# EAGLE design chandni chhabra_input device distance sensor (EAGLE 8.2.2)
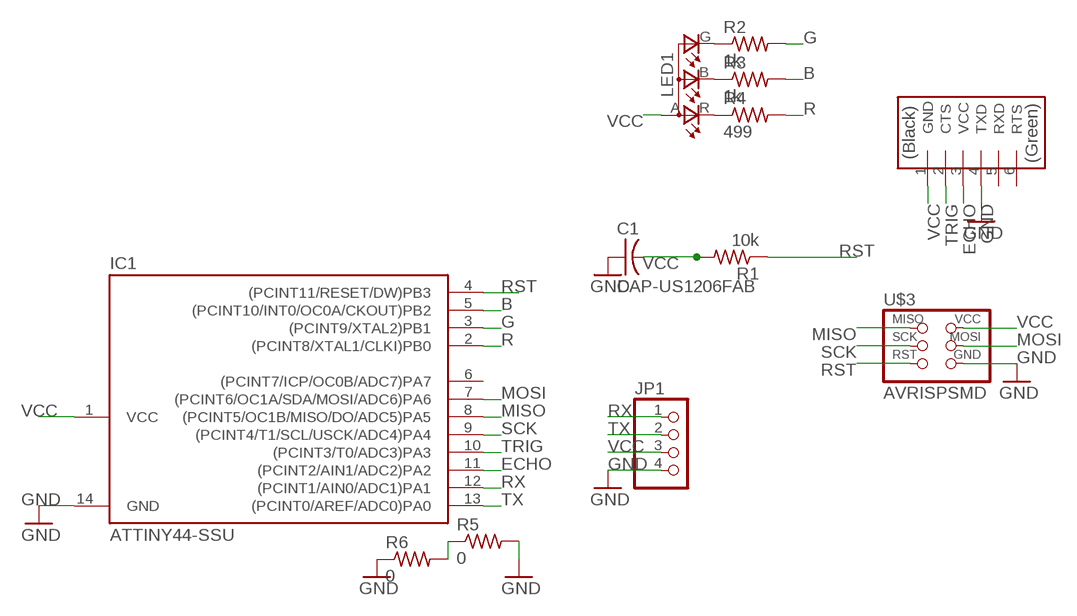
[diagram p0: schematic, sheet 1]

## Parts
C1  CAP-US1206FAB  [C1206FAB]
IC1  ATTINY44-SSU  [SOIC14]
JP1  PINHD-1X4  [1X04]
LED1  LEDRGBOLD  [P-LCC-4-3]
R1  10k  RES-US1206FAB  [R1206FAB]
R2  1k  RES-US1206FAB  [R1206FAB]
R3  1k  RES-US1206FAB  [R1206FAB]
R4  499  RES-US1206FAB  [R1206FAB]
R5  0  RES-US1206FAB  [R1206FAB]
R6  0  RES-US1206FAB  [R1206FAB]
U$1  FTDI-SMD-HEADER  [1X06SMD]
U$3  AVRISPSMD  [2X03SMD]

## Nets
B: IC1.5((PCINT10/INT0/OC0A/CKOUT)PB2) R3.2
ECHO: IC1.11((PCINT2/AIN1/ADC2)PA2) U$1.3(VCC)
G: IC1.3((PCINT9/XTAL2)PB1) R2.2
GND: C1.1 IC1.14(GND) JP1.4 R5.2 R6.1 U$1.4(TXD) U$3.6(GND)
MISO: IC1.8((PCINT5/OC1B/MISO/DO/ADC5)PA5) U$3.1(MISO)
MOSI: IC1.7((PCINT6/OC1A/SDA/MOSI/ADC6)PA6) U$3.4(MOSI)
N$1: R5.1 R6.2
N$2: LED1.G(CGREEN) R2.1
N$6: LED1.B(CBLUE) R3.1
N$7: LED1.R(CRED) R4.1
R: IC1.2((PCINT8/XTAL1/CLKI)PB0) R4.2
RST: IC1.4((PCINT11/RESET/DW)PB3) R1.1 U$3.5(RST)
RX: IC1.12((PCINT1/AIN0/ADC1)PA1) JP1.1
SCK: IC1.9((PCINT4/T1/SCL/USCK/ADC4)PA4) U$3.3(SCK)
TRIG: IC1.10((PCINT3/T0/ADC3)PA3) U$1.2(CTS)
TX: IC1.13((PCINT0/AREF/ADC0)PA0) JP1.2
VCC: C1.2 IC1.1(VCC) JP1.3 LED1.A(A2) R1.2 U$1.1(GND) U$3.2(VCC)
Unconnected: IC1.6((PCINT7/ICP/OC0B/ADC7)PA7) U$1.5(RXD) U$1.6(RTS)

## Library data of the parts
C1 = fab:CAP-US
IC1 = fab:ATTINY44
JP1 = pinhead:PINHD-1X4: PIN HEADER
LED1 = fab:LEDRGBOLD: OSRAM Hyper Multi TOPLED® Hyper-Bright LED LATB T686 Source: http://www.osram.convergy.de/
R1-R6 = fab:RES-US: Resistor (US Symbol)
U$1 = fab:FTDI-SMD-HEADER
U$3 = fab:AVRISP

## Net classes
0 default: width 0.035 mm, clearance 0.4 mm

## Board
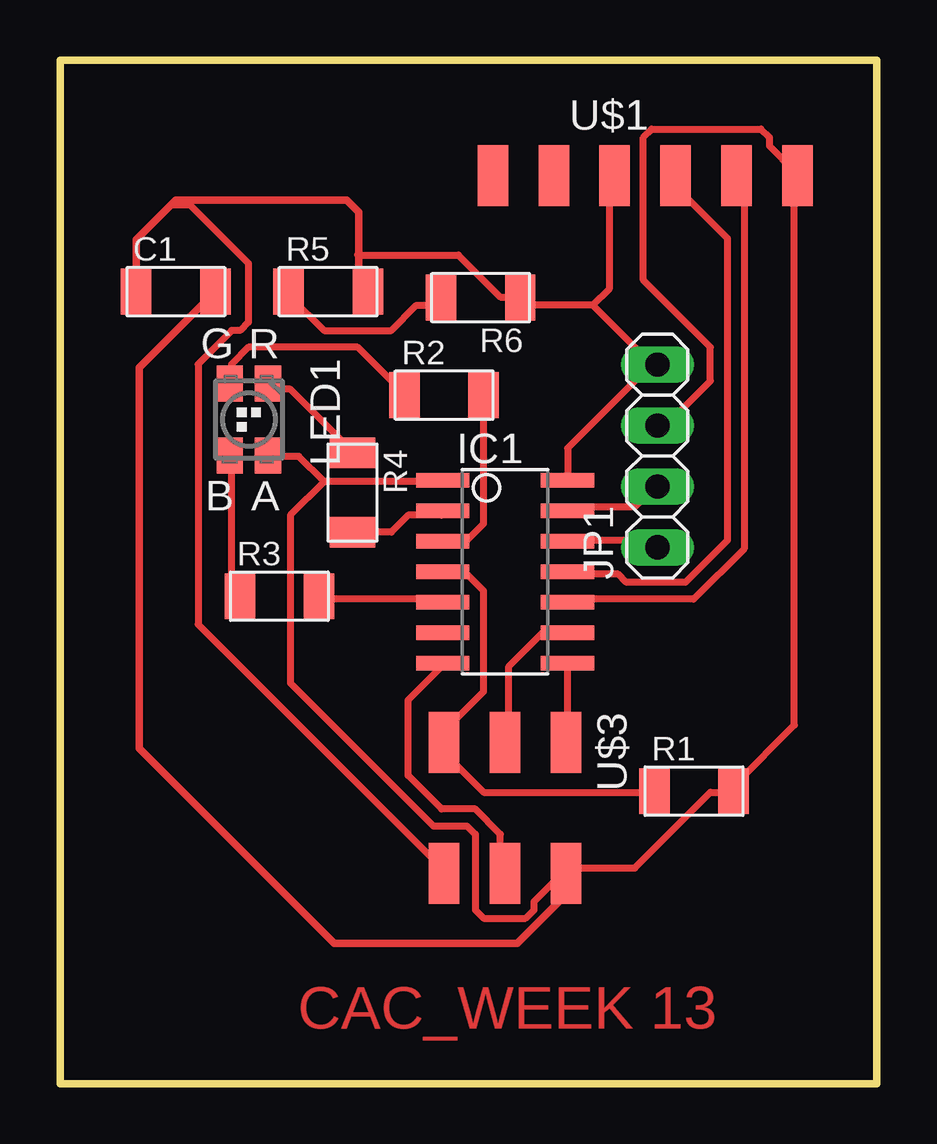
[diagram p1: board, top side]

Size 34.04 x 42.67 mm. Coordinates in mm from the lower left corner, seen from the top.
Outline: 34.04,42.67 0,42.67 0,0 34.04,0 34.04,42.67
Copper layers (1*16): Top 0.035mm / dielectric 1.5mm / Bottom 0.035mm
Design rules "fab": minimum track width 0.3mm, minimum drill 32mil, track to track 0.315mm, track to pad 0.315mm, pad to pad 0.315mm, via to via 0.315mm, smd to smd 0.315mm, copper to edge 40mil, drill to drill 16mil, minimum pad ring 10mil, minimum via ring 8mil, stop-mask expansion 4mil, vias tented up to drill 0mil, thermal gap 10mil

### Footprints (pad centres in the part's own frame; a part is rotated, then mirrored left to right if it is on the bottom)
C1206FAB = smd 1.27 x 1.905: 1 -1.651,0; 2 1.651,0
SOIC14 = smd 0.61 x 2.21: 1 -3.81,-2.603; 2 -2.54,-2.603; 3 -1.27,-2.603; 4 0,-2.603; 5 1.27,-2.603; 6 2.54,-2.603; 7 3.81,-2.603; 8 3.81,2.603; 9 2.54,2.603; 10 1.27,2.603; 11 0,2.603; 12 -1.27,2.603; 13 -2.54,2.603; 14 -3.81,2.603
1X04 = drill 1.016 long: 1 -3.81,0; 2 -1.27,0; 3 1.27,0; 4 3.81,0
P-LCC-4-3 = smd 1.1 x 1.5: A -0.8,1.5; B 0.8,1.5; G 0.8,-1.5; R -0.8,-1.5
R1206FAB = smd 1.27 x 1.905: 1 -1.651,0; 2 1.651,0
1X06SMD = smd 2.54 x 1.27: 1 0,6.35; 2 0,3.81; 3 0,1.27; 4 0,-1.27; 5 0,-3.81; 6 0,-6.35
2X03SMD = smd 2.54 x 1.27: 1 -2.54,2.54; 2 2.92,2.54; 3 -2.54,0; 4 2.92,0; 5 -2.54,-2.54; 6 2.92,-2.54

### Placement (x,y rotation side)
C1  4.83,33.02 0 top
IC1  18.54,21.34 270 top
JP1  24.89,26.16 90 top
LED1  7.87,27.69 180 top
R1  26.42,12.19 0 top
R2  16,28.7 0 top
R3  9.14,20.32 0 top
R4  12.19,24.64 270 top
R5  11.18,33.02 0 top
R6  17.53,32.77 180 top
U$1  24.38,37.85 270 top
U$3  18.54,11.68 270 top

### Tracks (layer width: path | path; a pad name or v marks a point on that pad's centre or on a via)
B
  Top 0.3: R3.2 11,20.19 15.9,20.19 IC1.5
ECHO
  Top 0.3: IC1.11 21.15,21.24 23.25,21.24 23.6,20.89 26.05,20.89 27.8,22.64 27.8,35.24 25.35,37.69 U$1.3
G
  Top 0.3: R2.2 17.65,28.59 17.65,23.34 16.95,22.64 16.25,22.64 IC1.3
GND
  Top 0.3: 22.2,32.44 19.4,32.44 R6.1 19.05,32.79 18.35,32.79 16.6,34.54 12.45,34.54 12.4,34.54 | 24.65,29.99 22.2,32.44 | 24.65,29.99 21.15,26.49 21.15,25.44 IC1.14 | 24.65,29.99 JP1.4 | 22.2,32.44 22.9,33.14 22.9,37.69 U$1.4 | U$3.6 15.9,8.99 5.75,19.14 5.75,29.99 7.15,31.39 7.5,31.39 7.85,31.74 7.85,34.19 5.4,36.64 4.7,36.64 4.67,36.68
  Top 0.305: C1.1 3.17,35.18 4.67,36.68 4.83,36.83 11.94,36.83 12.45,36.32 12.45,34.54 12.45,33.4 R5.2
MISO
  Top 0.3: IC1.8 21.15,17.39 21.15,14.24 U$3.1
MOSI
  Top 0.3: IC1.7 15.9,17.39 14.5,15.99 14.5,12.84 15.9,11.44 17.3,11.44 18.35,10.39 18.35,8.99 U$3.4
N$1
  Top 0.3: R6.2 15.55,32.44 14.85,32.44 13.8,31.39 11,31.39 9.6,32.79 R5.1
N$2
  Top 0.3: LED1.G 7.15,29.29 7.15,29.99 7.85,30.69 12.4,30.69 14.15,28.94 R2.1
N$6
  Top 0.3: LED1.B 7.15,26.14 7.15,20.54 R3.1
N$7
  Top 0.3: LED1.R 8.9,28.94 9.6,28.94 12.05,26.49 R4.1
R
  Top 0.3: R4.2 12.4,22.99 13.8,22.99 14.5,23.69 15.9,23.69 IC1.2
RST
  Top 0.3: R1.1 24.65,12.14 17.65,12.14 15.9,13.89 U$3.5 16.25,14.24 16.25,14.94 17.65,16.34 17.65,20.54 16.95,21.24 16.25,21.24 IC1.4
RX
  Top 0.3: IC1.12 21.15,22.64 24.65,22.64 JP1.1
SCK
  Top 0.3: IC1.9 20.8,18.79 20.1,18.79 18.7,17.39 18.7,14.24 U$3.3
TRIG
  Top 0.3: IC1.10 21.15,20.19 26.4,20.19 28.5,22.29 28.5,37.69 U$1.2
TX
  Top 0.3: IC1.13 21.15,24.04 23.95,24.04 24.65,24.74 JP1.2
VCC
  Top 0.3: JP1.3 25,27.19 27.1,29.29 27.1,30.69 24.3,33.49 24.3,39.44 24.65,39.79 29.2,39.79 29.55,39.44 29.55,39.09 30.6,38.04 U$1.1 30.6,37.69 30.6,14.94 28.15,12.49 R1.2 27.8,12.14 27.1,12.14 23.95,8.99 21.15,8.99 U$3.2 20.8,8.64 19.75,7.59 19.75,7.24 19.4,6.89 17.65,6.89 17.3,7.24 17.3,10.39 16.95,10.74 15.55,10.74 9.6,16.69 9.6,23.69 11,25.09 | 11,25.09 9.95,26.14 8.9,26.14 LED1.A | 11,25.09 15.9,25.09 IC1.1
  Top 0.305: C1.2 3.3,29.84 3.3,13.97 11.43,5.84 19.05,5.84 21.08,7.87 U$3.2

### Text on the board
Top: CAC_WEEK 13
